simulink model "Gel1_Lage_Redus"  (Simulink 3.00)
settings: Solver=ode5  SolverMode=SingleTasking  StartTime=0.0  StopTime=1.75  RelTol=1e-3  AbsTol=1e-6
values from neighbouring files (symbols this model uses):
  alpha = 2*dR*TR*KI-(1/K_St)    [Red_Par.m]
  beta = 0    [Red_Par.m]
  bm = 4    [PI_Par.m]    (also in Red_Par.m)
  K_St = 1/FD_Stern    (= 2.27848101266)    [PI_Par.m]    (also in Red_Par.m = 1/FD_Stern)
  KI = T_St_max/(K_St*TR^2)    [Red_Par.m]
  KL = omd*sqrt((1-TR^2*omd^2)+4*dR^2*TR^2*omd^2)    [PI_Par.m]    (also in Red_Par.m)
  KVor = 1    [PI_Par.m]    (also in Red_Par.m)
  qA = 0    [PI_Par.m]    (also in Red_Par.m)
  T_St = M_Stern/FD_Stern    (= 2.82860759494)    [PI_Par.m]    (also in Red_Par.m = M_Stern/FD_Stern)
  tb = vm/bm    (= 0.5)    [PI_Par.m]    (also in Red_Par.m)
  te = tv+tb    (= 1.2853981634)    [PI_Par.m]    (also in Red_Par.m)
  tv = se/vm    (= 0.785398163397)    [PI_Par.m]    (also in Red_Par.m)
  Vorz = 1    [PI_Par.m]    (also in Red_Par.m)
  z0 = (1/KM)*(rh)    (= 1.25)    [PI_Par.m]    (also in Red_Par.m = (1/KM)*(rh))

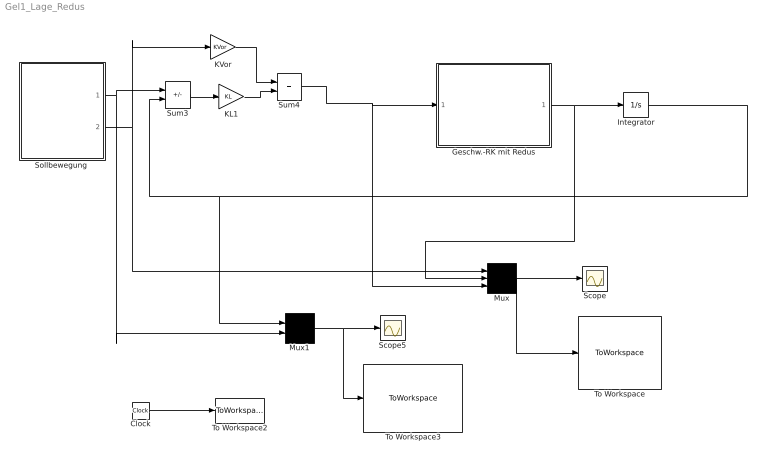
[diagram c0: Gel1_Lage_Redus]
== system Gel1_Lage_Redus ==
  Clock : Clock
  Geschw.-RK mit Redus : Subsystem
  Integrator : Integrator  ExternalReset=none  InitialConditionSource=internal  InitialCondition=0  LimitOutput=off  UpperSaturationLimit=inf  LowerSaturationLimit=-inf  ShowSaturationPort=off  ShowStatePort=off  AbsoluteTolerance=auto
  KL1 : Gain  Gain=KL  SaturateOnIntegerOverflow=on
  KVor : Gain  Gain=KVor  SaturateOnIntegerOverflow=on
  Mux : Mux  Inputs=3
  Mux1 : Mux  Inputs=2
  Scope : Scope
  Scope5 : Scope
  "Sollbewegung " : Subsystem
  Sum3 : Sum  Inputs=+-  SaturateOnIntegerOverflow=on
  Sum4 : Sum  Inputs=++  SaturateOnIntegerOverflow=on
  To Workspace : ToWorkspace  VariableName=Geschw_Red_M_Quer  SampleTime=0.001  SaveFormat=Matrix
  To Workspace2 : ToWorkspace  VariableName=Zeit_Lage  SampleTime=0.001  SaveFormat=Matrix
  To Workspace3 : ToWorkspace  VariableName=Lage_Red_M_Quer  SampleTime=0.001  SaveFormat=Matrix
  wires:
  Sum3/1 -> KL1/1
  KL1/1 -> Sum4/2
  KVor/1 -> Sum4/1
  Mux/1 -> To Workspace/1, Scope/1
  "Sollbewegung "/2(qpss) -> KVor/1, Mux/1
  Geschw.-RK mit Redus/1(v) -> Integrator/1, Mux/2
  Sum4/1 -> Geschw.-RK mit Redus/1(vs), Mux/3
  Mux1/1 -> To Workspace3/1, Scope5/1
  "Sollbewegung "/1(qS) -> Sum3/1, Mux1/2
  Integrator/1 -> Sum3/2, Mux1/1
  Clock/1 -> To Workspace2/1

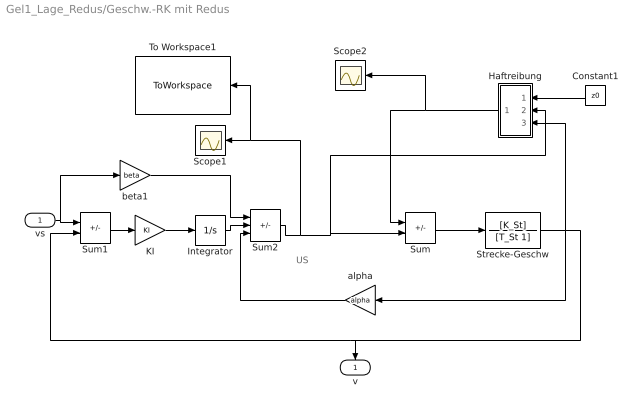
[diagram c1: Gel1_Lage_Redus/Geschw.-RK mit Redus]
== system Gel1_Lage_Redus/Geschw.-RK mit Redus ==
  note: US
  vs : Inport  Port=1  PortWidth=-1  SampleTime=-1  DataType=auto
  Constant1 : Constant  Orientation=left  Value=z0
  Haftreibung : Subsystem  Orientation=left
  Integrator : Integrator  ExternalReset=none  InitialConditionSource=internal  InitialCondition=0  LimitOutput=off  UpperSaturationLimit=inf  LowerSaturationLimit=-inf  ShowSaturationPort=off  ShowStatePort=off  AbsoluteTolerance=auto
  KI : Gain  Gain=KI  SaturateOnIntegerOverflow=on
  Scope1 : Scope
  Scope2 : Scope
  Strecke-Geschw : TransferFcn  Numerator=[K_St]  Denominator=[T_St 1]
  Sum : Sum  Inputs=-+  SaturateOnIntegerOverflow=on
  Sum1 : Sum  Inputs=+-  SaturateOnIntegerOverflow=on
  Sum2 : Sum  Inputs=++-  SaturateOnIntegerOverflow=on
  To Workspace1 : ToWorkspace  VariableName=Red_M_Quer_US  SampleTime=0.001  SaveFormat=Matrix
  alpha : Gain  Orientation=left  Gain=alpha  SaturateOnIntegerOverflow=on
  beta1 : Gain  Gain=beta  SaturateOnIntegerOverflow=on
  v : Outport  Orientation=down  Port=1
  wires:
  Strecke-Geschw/1 -> Haftreibung/3(qp), alpha/1, Sum1/2, v/1
  Sum/1 -> Strecke-Geschw/1
  Constant1/1 -> Haftreibung/1(z0)
  Haftreibung/1(Out1) -> Sum/1, Scope2/1
  Sum1/1 -> KI/1
  KI/1 -> Integrator/1
  Sum2/1 -> Sum/2, Haftreibung/2(US), Scope1/1, To Workspace1/1
  Integrator/1 -> Sum2/2
  alpha/1 -> Sum2/3
  beta1/1 -> Sum2/1
  vs/1 -> Sum1/1, beta1/1

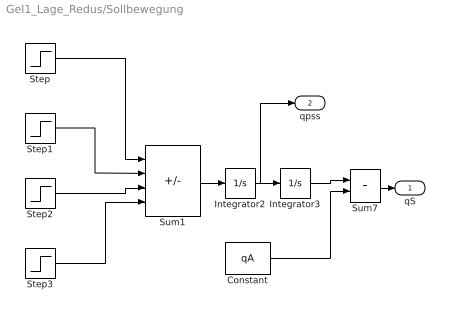
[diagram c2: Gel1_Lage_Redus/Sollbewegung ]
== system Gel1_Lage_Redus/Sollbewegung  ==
  Constant : Constant  Value=qA
  Integrator2 : Integrator  ExternalReset=none  InitialConditionSource=internal  InitialCondition=0  LimitOutput=off  UpperSaturationLimit=inf  LowerSaturationLimit=-inf  ShowSaturationPort=off  ShowStatePort=off  AbsoluteTolerance=auto
  Integrator3 : Integrator  ExternalReset=none  InitialConditionSource=internal  InitialCondition=0  LimitOutput=off  UpperSaturationLimit=inf  LowerSaturationLimit=-inf  ShowSaturationPort=off  ShowStatePort=off  AbsoluteTolerance=auto
  Step : Step  Time=0  Before=0  After=bm*Vorz  SampleTime=0.005
  Step1 : Step  Time=tb  Before=0  After=bm*Vorz  SampleTime=0.005
  Step2 : Step  Time=tv  Before=0  After=bm*Vorz  SampleTime=0.005
  Step3 : Step  Time=te  Before=0  After=bm*Vorz  SampleTime=0.005
  Sum1 : Sum  Inputs=+--+  SaturateOnIntegerOverflow=on
  Sum7 : Sum  Inputs=++  SaturateOnIntegerOverflow=on
  qS : Outport  Port=1  InitialOutput=0
  qpss : Outport  Port=2
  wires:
  Step/1 -> Sum1/1
  Step1/1 -> Sum1/2
  Step2/1 -> Sum1/3
  Step3/1 -> Sum1/4
  Sum1/1 -> Integrator2/1
  Integrator2/1 -> Integrator3/1, qpss/1
  Constant/1 -> Sum7/2
  Integrator3/1 -> Sum7/1
  Sum7/1 -> qS/1

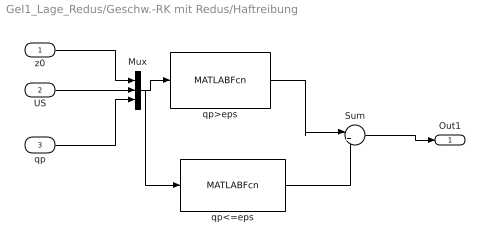
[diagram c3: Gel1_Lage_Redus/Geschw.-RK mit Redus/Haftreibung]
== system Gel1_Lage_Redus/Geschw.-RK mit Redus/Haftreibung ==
  z0 : Inport  Port=1  PortWidth=-1  SampleTime=-1  DataType=auto
  US : Inport  Port=2  PortWidth=-1  SampleTime=-1  DataType=auto
  qp : Inport  Port=3  PortWidth=-1  SampleTime=-1  DataType=auto
  Mux : Mux  Inputs=3
  Sum : Sum  Inputs=|++  SaturateOnIntegerOverflow=on
  qp<=eps : MATLABFcn  MATLABFcn=(abs(u(3)) < eps) *min(abs(u(2)),u(1))* sign(u(2))*sign(u(1))  OutputWidth=1  OutputSignalType=auto
  qp>eps : MATLABFcn  MATLABFcn=(abs(u(3)) > eps) * sign(u(3))*u(1)  OutputWidth=1  OutputSignalType=auto
  Out1 : Outport  Port=1  InitialOutput=0
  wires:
  z0/1 -> Mux/1
  US/1 -> Mux/2
  qp/1 -> Mux/3
  Mux/1 -> qp>eps/1, qp<=eps/1
  Sum/1 -> Out1/1
  qp>eps/1 -> Sum/1
  qp<=eps/1 -> Sum/2
